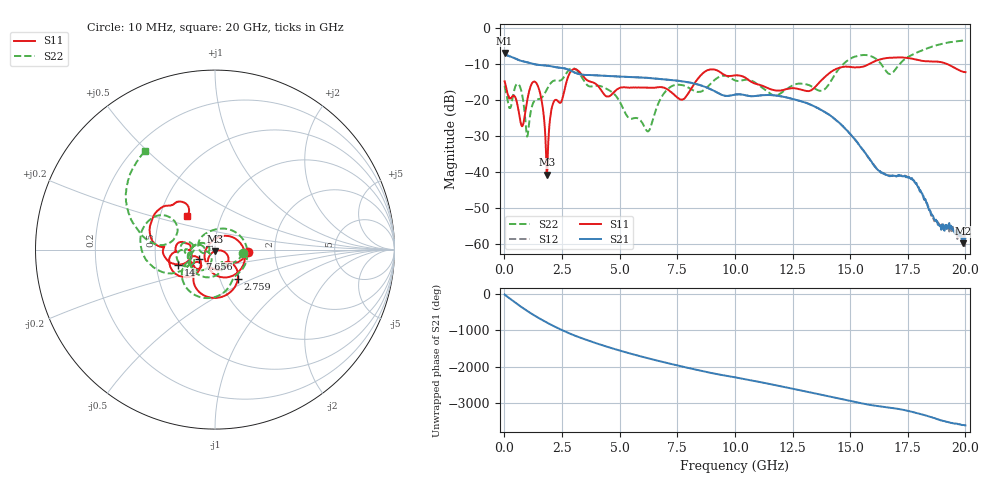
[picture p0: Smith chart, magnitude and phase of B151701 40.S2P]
!  2-Port S-parameters saved by WinCal
! VAR MeasName=S-Parameters (CALIBRATED_DATA) read from VNA (N5244A)
! VAR MeasDate=2015-12-24 19:14:04
! VAR NAME=B151701 40
! VAR FILENAME=B151701 40.S2P
! VAR DATE=2015-12-24 19:14:04
! VAR PHYS_PORTS=1,3
# Hz S DB R 50
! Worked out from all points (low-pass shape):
!   801 points, 10 MHz to 20 GHz, reference 50 ohm
!   highest |S21| = -6.90 dB at 10 MHz (marker M1); lowest = -59.7 dB at 19.9 GHz (marker M2)
!   |S21| within 3 dB of the highest: start of sweep to 1.192 GHz
!   lowest |S11| = -40.7 dB at 1.834 GHz (marker M3), VSWR 1.02, Z = 49.8 - j0.903 ohm
!   |S11| at or under -10 dB: start of sweep to 15.83 GHz; 19.19 GHz to end of sweep
!   |S22| runs from -30.1 to -3.5 dB; largest |S21 - S12| = 0.0014
!   S11 on the Smith chart (normalised r, x): 10 MHz: 1.44, -0.05; 2.759 GHz: 1.21, -0.42; 7.656 GHz: 0.83, -0.09; 14 GHz: 0.65, -0.11; 20 GHz: 0.69, +0.27
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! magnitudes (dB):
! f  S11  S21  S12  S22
! 10 MHz  -14.8  -6.9  -6.9  -16.1
! 759.6 MHz  -27.2  -9.2  -9.2  -18.1
! 1.01 GHz  -19.5  -9.6  -9.6  -29.9
! 1.384 GHz  -15.3  -10.2  -10.2  -19.8
! 1.834 GHz  -40.7  -10.4  -10.4  -17.1
! 2.109 GHz  -21.0  -10.7  -10.7  -14.7
! 2.759 GHz  -13.6  -11.5  -11.5  -11.9
! 3.358 GHz  -13.0  -12.9  -12.9  -13.7
! 4.458 GHz  -19.0  -13.3  -13.3  -17.0
! 6.207 GHz  -16.6  -13.8  -13.8  -28.7
! 6.682 GHz  -16.5  -14.1  -14.1  -20.9
! 7.656 GHz  -19.8  -14.7  -14.7  -15.8
! 8.806 GHz  -11.7  -16.6  -16.5  -16.4
! 10.01 GHz  -13.2  -18.5  -18.5  -14.5
! 13.35 GHz  -17.1  -21.5  -21.5  -16.3
! 14 GHz  -13.1  -23.7  -23.8  -16.2
! 15.38 GHz  -10.9  -32.3  -32.3  -7.7
! 16.68 GHz  -8.3  -41.0  -40.8  -12.7
! 17.68 GHz  -8.5  -41.6  -41.8  -7.5
! 18.73 GHz  -9.3  -53.2  -53.6  -4.8
! 19.9 GHz  -12.2  -59.7  -57.9  -3.5
! 20 GHz  -12.3  -58.3  -59.8  -3.5
